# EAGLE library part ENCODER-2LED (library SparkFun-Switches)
Illuminated Rotary Encoder w/ 2 LEDs Rotary encoders rotate similarly to potentiometers, but they’re different from potentiometers in that an encoder has full rotation without limits. They output gray code so that you can tell how much and in which direction the encoder has been turned. This encoder has a red/green LED built-in, which shines through the encoder shaft. SparkFun Products Rotary Encoder - Illuminated (Red/Green) (COM-10596) SparkFun Rotary Encoder Breakout - Illuminated (RG/RGB) (BOB-11722)
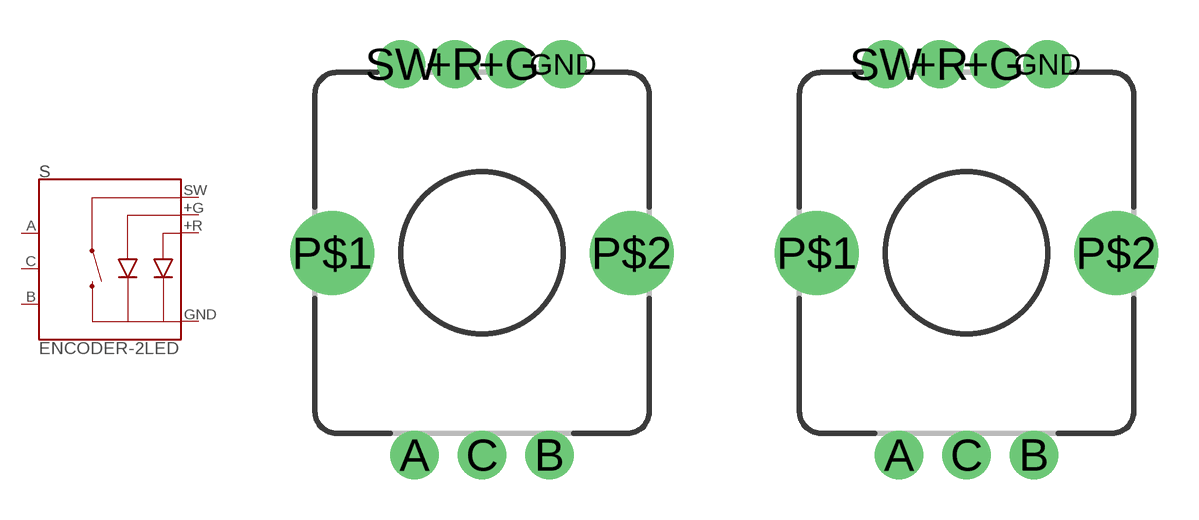
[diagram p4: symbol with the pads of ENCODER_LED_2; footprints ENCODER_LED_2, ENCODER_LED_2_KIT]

Designator prefix S

## ENCODER-2LED (PROD_ID: COMP-11113; SF_SKU: COM-10596)  [ENCODER_LED_2]
+G  +G  pas
+R  +R  pas
A  A
B  B
C  C
GND  -  pas
SW  SW  pas

## ENCODER-2LEDKIT (PROD_ID: COMP-11113; SF_SKU: COM-10596)  [ENCODER_LED_2_KIT]
Pads as for ENCODER_LED_2

## Footprint ENCODER_LED_2 (pad centres in mm)
Illuminated Rotary Encoder w/ 2 LEDs Rotary encoders rotate similarly to potentiometers, but they’re different from potentiometers in that an encoder has full rotation without limits. They output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
drill 1.1 pad 1.778: +G 1,7; +R -1,7; GND 3,7; SW -3,7
drill 1.1 pad 1.8: A -2.5,-7.5; B 2.5,-7.5; C 0,-7.5
drill 2.1: P$1 -5.55,0; P$2 5.55,0

## Footprint ENCODER_LED_2_KIT (pad centres in mm)
Illuminated Rotary Encoder w/ 2 LEDs - KIT Package Rotary encoders rotate similarly to potentiometers, but they’re different from potentiometers in that an encoder has full rotation without limits.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
drill 1.1 pad 1.778: +G 1,7; +R -1,7; GND 3,7; SW -3,7
drill 1.1 pad 1.8: A -2.5,-7.5; B 2.5,-7.5; C 0,-7.5
drill 2.1: P$1 -5.55,0; P$2 5.55,0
